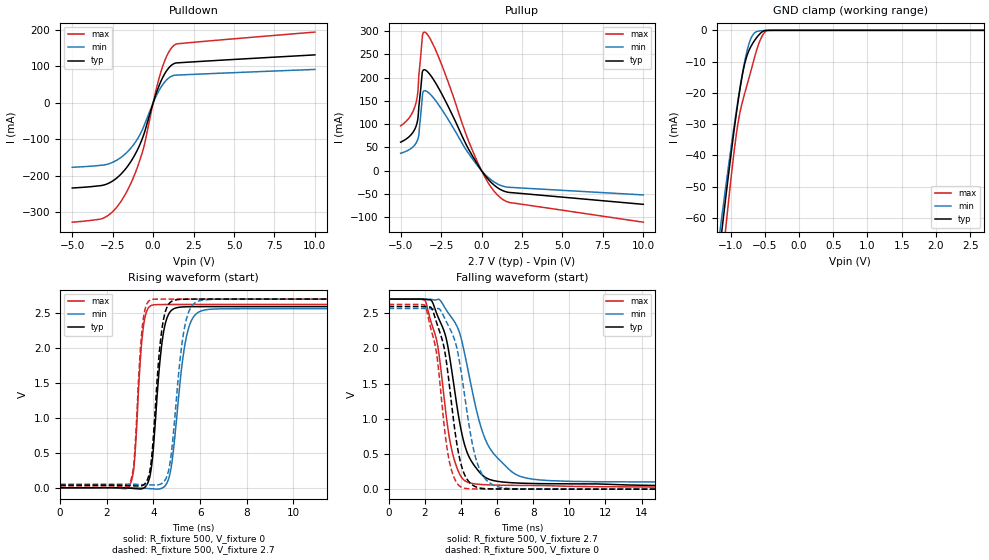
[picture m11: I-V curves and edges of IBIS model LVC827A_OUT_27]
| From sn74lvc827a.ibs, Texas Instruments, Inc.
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[Model]   LVC827A_OUT_27
Model_type  3-state
Enable   Active-Low
Vref =   0
Rref =   500
Cref =   50p
Vmeas =   1.5
| variable   typ   min   max
C_comp   5.87pF   5.21pF   6.89pF
| C_pullup   7.39pF   6.53pF   8.04pF
| C_pulldown   10.34pF   7.04pF   16.10pF
| C_tri-state   5.87pF   5.21pF   6.89pF
[Temperature Range]   40   100   -40
| Ambient temperature   25   85   -40
[Voltage range]   2.7   2.7   2.7
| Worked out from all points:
|   slope of the pulldown table from 0 to 0.405 V, typ, clamps not added: 7.86 ohm
|   slope of the pullup table from 0 to 0.405 V, typ, clamps not added: 22.2 ohm
|   GND clamp passes 1 mA (typ) near -0.57 V on its own axis
|   rising waveform, R_fixture 500, V_fixture 0: 20-80 % time 381ps typ, 503ps min, 283ps max; typ from 0 V to 2.59 V
|   falling waveform, R_fixture 500, V_fixture 2.7: 20-80 % time 1.12ns typ, 1.62ns min, 881ps max; typ from 2.7 V to 0.037 V
|   rising waveform, R_fixture 500, V_fixture 2.7: 20-80 % time 365ps typ, 474ps min, 274ps max; typ from 0.037 V to 2.7 V
|   falling waveform, R_fixture 500, V_fixture 0: 20-80 % time 851ps typ, 1.02ns min, 742ps max; typ from 2.6 V to 0 V
[GND Clamp]
| LVC827A_OUT_27
|   Voltage   I(typ)   I(min)   I(max)
-5V       -931.5mA   -844.2mA   -1.078A
-1.165V   -71.26mA   -65.92mA   -83.86mA
-1.13V    -64.59mA   -59.94mA   -76.11mA
-1.065V   -52.46mA   -49.07mA   -62.05mA
-910mV    -25.74mA   -24.94mA   -32.36mA
-865mV    -19.06mA   -18.67mA   -26.5mA
-790mV    -10.37mA   -9.555mA   -19.88mA
-730mV    -6.383mA   -4.223mA   -15.17mA
-670mV    -3.933mA   -1.323mA   -10.3mA
-565mV    -979.4uA   -160.5uA   -3.019mA
-480mV    -15.61uA   -59.52uA   -228.3uA
2.7V      68.83pA    197.5pA    704.9pA
[Pulldown]
| LVC827A_OUT_27
|   Voltage   I(typ)   I(min)   I(max)
-5V       -233.6mA   -176.7mA   -327.5mA
-2.98V    -224.5mA   -169.9mA   -314.3mA
-2.365V   -210.1mA   -160.1mA   -292.1mA
-1.755V   -183.9mA   -141.2mA   -253.6mA
-1.17V    -145.7mA   -112.3mA   -199.5mA
-645mV    -95.11mA   -71.31mA   -132.2mA
-490mV    -74.32mA   -54.49mA   -105mA
150mV     20.96mA    15.3mA     30.02mA
550mV     66.02mA    47.72mA    95.08mA
920mV     93.69mA    66.9mA     135.9mA
1.29V     107.9mA    75.7mA     158.1mA
10V       131.9mA    91.98mA    194.5mA
[Pullup]
| LVC827A_OUT_27
|   Voltage   I(typ)   I(min)   I(max)
-5V       61.13mA    37.23mA    96.09mA
-4.41V    75.09mA    46.34mA    116.6mA
-4.06V    94.28mA    58.44mA    144.5mA
-3.94V    110.7mA    67.31mA    168.4mA
-3.875V   137.7mA    77.24mA    205.2mA
-3.65V    212.9mA    162.4mA    290.5mA
-3.5V     216.5mA    171.7mA    297.4mA
-2.605V   174.2mA    139.1mA    239.9mA
-245mV    13.35mA    10.56mA    18.11mA
450mV     -20.03mA   -15.76mA   -28.31mA
1.125V    -39.79mA   -30.95mA   -56.95mA
10V       -72.48mA   -52.25mA   -110.8mA
[Ramp]
| LVC827A_OUT_27
| variable   typ   min   max
dV/dt_r   1.57/3.91E-10   1.55/5.07E-10   1.58/2.97E-10
dV/dt_f   1.60/1.12E-09   1.59/1.62E-09   1.60/8.85E-10
R_load = 500
[Rising Waveform]
| LVC827A_OUT_27
R_fixture =   500
C_fixture =   0
L_fixture =   0
V_fixture =   0
V_fixture_min = 0
V_fixture_max = 0
|   Time   V(typ)   V(min)   V(max)
0s        507.6pV    2.115nV    14.6nV
2.985ns   -6.257mV   1.02mV     37.83mV
3.18ns    -11.29mV   -99.3uV    357.6mV
3.57ns    -6.454mV   -6.863mV   2.306V
4.005ns   600.7mV    -16.17mV   2.617V
4.31ns    1.916V     -12.4mV    2.621V
4.59ns    2.44V      76.77mV    2.622V
5.42ns    2.59V      2.171V     2.623V
6.23ns    2.592V     2.546V     2.623V
50ns      2.592V     2.563V     2.623V
[Falling Waveform]
| LVC827A_OUT_27
R_fixture =   500
C_fixture =   0
L_fixture =   0
V_fixture =   2.7
V_fixture_min = 2.7
V_fixture_max = 2.7
|   Time   V(typ)   V(min)   V(max)
0s        2.7V       2.7V       2.7V
2.01ns    2.697V     2.7V       2.685V
2.43ns    2.656V     2.693V     2.313V
3.15ns    2.182V     2.563V     1.13V
3.54ns    1.61V      2.419V     509.7mV
4.07ns    772.1mV    2.087V     157.8mV
4.585ns   397mV      1.452V     82.92mV
5.67ns    131.3mV    554.4mV    59.6mV
8.065ns   80.23mV    139.2mV    52.55mV
50ns      36.67mV    50.41mV    25.63mV
[Rising Waveform]
| LVC827A_OUT_27
R_fixture =   500
C_fixture =   0
L_fixture =   0
V_fixture =   2.7
V_fixture_min = 2.7
V_fixture_max = 2.7
|   Time   V(typ)   V(min)   V(max)
0s        36.62mV    50.05mV    25.63mV
2.98ns    30.96mV    50.81mV    68.55mV
3.17ns    27.47mV    49.76mV    384.3mV
3.535ns   33.57mV    44.47mV    2.338V
3.925ns   446.7mV    40.45mV    2.694V
4.26ns    1.966V     47.24mV    2.699V
4.52ns    2.531V     122.3mV    2.7V
5.35ns    2.698V     2.322V     2.7V
6.09ns    2.7V       2.686V     2.7V
50ns      2.7V       2.7V       2.7V
[Falling Waveform]
| LVC827A_OUT_27
R_fixture =   500
C_fixture =   0
L_fixture =   0
V_fixture =   0
V_fixture_min = 0
V_fixture_max = 0
|   Time   V(typ)   V(min)   V(max)
0s        2.595V     2.567V     2.625V
1.98ns    2.593V     2.567V     2.618V
2.43ns    2.547V     2.561V     2.196V
3.05ns    2.04V      2.458V     969.6mV
3.365ns   1.478V     2.294V     394.5mV
3.8ns     613.6mV    1.982V     80.21mV
4.205ns   206.5mV    1.338V     13.19mV
5.045ns   16.49mV    278.1mV    2.626mV
6.455ns   2.096mV    13.38mV    910.4uV
50ns      17.4uV     76.42uV    5.402uV
